
DATA_BLOCK DB3401
TITLE=
VERSION : 0.1

STRUCT
   CM_ID : STRING  [8 ] := '=CSF'; //COMPOSITE MACHINE
   STATION_ID : STRING  [8 ] := '++OP40'; //STATION - TRATTO - ZONE
   ELEMENT_ID : STRING  [8 ] := '+CAB0'; //ELEMENT
   DB_ID : INT := 0 ; //DB SIZE OR TYPE
   PART_STYLE : STRING  [12 ]; //PART STYLE ON LAST STATION
   ACT_CYCLE_TIME : INT ; //ACTUAL CYCLE TIME FOR THIS STYLE
   COUNT_GOOD : INT ; //COUNTER GOOD PIECES
   COUNT_SCRAP : INT ; //COUNTER SCRAP PIECES
   SPARE_00 : ARRAY  [0 .. 15 ] OF //SPARE INTEGER
   INT ;
   SPARE_01 : ARRAY  [0 .. 17 ] OF //SPARE INTEGER
   INT ;
   CODE_EVENT : ARRAY  [0 .. 7 ] OF //CODE EVENT - EXTENDED FAULT CODE DIAGNOSTIC
   INT ;
   EVENT : STRUCT
E0000 : BOOL ; //+CAB0-0ESP10_Q1; 0ESP10_Q1;1
E0001 : BOOL ; //+CAB0-0ESP10_Q2; 0ESP10_Q2;1
E0002 : BOOL ; //+CAB0-0ESP10_0F1; 0ESP10_0F1;1
E0003 : BOOL ; //+CAB0-0ESP10_0F2; 0ESP10_0F2;1
E0004 : BOOL ; //+CAB0-0ESP10_0F3; 0ESP10_0F3;1
E0005 : BOOL ; //+CAB0-0DC43_Q1; 0DC43_Q1;1
E0006 : BOOL ; //+CAB0-0DC43_F1; 0DC43_F1;1
E0007 : BOOL ; //+CAB0-0DC44_UPS; 0DC44_UPS;1
E0008 : BOOL ; //+CAB0-0DC44_0F1; 0DC44_0F1;1
E0009 : BOOL ; //+CAB0-0DP58_A1; 0DP58_A1;1
E0010 : BOOL ; //+CAB0-0EN64_S1F; 0EN64_S1F;1
E0011 : BOOL ; //+CAB0-0FIP65_Q1; 0FIP65_Q1;1
E0012 : BOOL ; //+CAB0-0SPS90_A1; 0SPS90_A1;1
E0013 : BOOL ; //+CAB0-0SPS91_D1; 0SPS91_D1;1
E0014 : BOOL ; //+CAB0-0SPS92_A1; 0SPS92_A1;1
E0015 : BOOL ; //+CAB0-0SPS92_A2; 0SPS92_A2;1
E0016 : BOOL ; //+CAB0-0SPS93_A1; 0SPS93_A1;1
E0017 : BOOL ; //+CAB0-0SPS93_A2; 0SPS93_A2;1
E0018 : BOOL ; //+CAB0-0SPS93_A3; 0SPS93_A3;1
E0019 : BOOL ; //+CAB0-0SPS93_A4; 0SPS93_A4;1
E0020 : BOOL ; //+CAB0-0SPS93_A5; 0SPS93_A5;1
E0021 : BOOL ; //+CAB0-0SPS93_A6; 0SPS93_A6;1
E0022 : BOOL ; //+CAB0-0SPS93_A7; 0SPS93_A7;1
E0023 : BOOL ; //+CAB0-0SPS93_A8; 0SPS93_A8;1
E0024 : BOOL ; //+CAB0-0SPS93_A9; 0SPS93_A9;1
E0025 : BOOL ;
E0026 : BOOL ;
E0027 : BOOL ;
E0028 : BOOL ;
E0029 : BOOL ;
E0030 : BOOL ;
E0031 : BOOL ;
E0032 : BOOL ;
E0033 : BOOL ;
E0034 : BOOL ;
E0035 : BOOL ;
E0036 : BOOL ;
E0037 : BOOL ;
E0038 : BOOL ;
E0039 : BOOL ;
E0040 : BOOL ;
E0041 : BOOL ;
E0042 : BOOL ;
E0043 : BOOL ;
E0044 : BOOL ;
E0045 : BOOL ;
E0046 : BOOL ;
E0047 : BOOL ;
E0048 : BOOL ;
E0049 : BOOL ;
E0050 : BOOL ;
E0051 : BOOL ;
E0052 : BOOL ;
E0053 : BOOL ;
E0054 : BOOL ;
E0055 : BOOL ;
E0056 : BOOL ;
E0057 : BOOL ;
E0058 : BOOL ;
E0059 : BOOL ;
E0060 : BOOL ;
E0061 : BOOL ;
E0062 : BOOL ;
E0063 : BOOL ;
   END_STRUCT;
END_STRUCT;
BEGIN
CM_ID := '=CSF';
STATION_ID := '++OP40';
ELEMENT_ID := '+CAB0';
DB_ID := 0 ;
PART_STYLE := '';
ACT_CYCLE_TIME := 0;
COUNT_GOOD := 0;
COUNT_SCRAP := 0;
SPARE_00[0] := 0;
SPARE_00[1] := 0;
SPARE_00[2] := 0;
SPARE_00[3] := 0;
SPARE_00[4] := 0;
SPARE_00[5] := 0;
SPARE_00[6] := 0;
SPARE_00[7] := 0;
SPARE_00[8] := 0;
SPARE_00[9] := 0;
SPARE_00[10] := 0;
SPARE_00[11] := 0;
SPARE_00[12] := 0;
SPARE_00[13] := 0;
SPARE_00[14] := 0;
SPARE_00[15] := 0;
SPARE_01[0] := 0;
SPARE_01[1] := 0;
SPARE_01[2] := 0;
SPARE_01[3] := 0;
SPARE_01[4] := 0;
SPARE_01[5] := 0;
SPARE_01[6] := 0;
SPARE_01[7] := 0;
SPARE_01[8] := 0;
SPARE_01[9] := 0;
SPARE_01[10] := 0;
SPARE_01[11] := 0;
SPARE_01[12] := 0;
SPARE_01[13] := 0;
SPARE_01[14] := 0;
SPARE_01[15] := 0;
SPARE_01[16] := 0;
SPARE_01[17] := 0;
CODE_EVENT[0] := 0;
CODE_EVENT[1] := 0;
CODE_EVENT[2] := 0;
CODE_EVENT[3] := 0;
CODE_EVENT[4] := 0;
CODE_EVENT[5] := 0;
CODE_EVENT[6] := 0;
CODE_EVENT[7] := 0;
EVENT.E0000 := FALSE;
EVENT.E0001 := FALSE;
EVENT.E0002 := FALSE;
EVENT.E0003 := FALSE;
EVENT.E0004 := FALSE;
EVENT.E0005 := FALSE;
EVENT.E0006 := FALSE;
EVENT.E0007 := FALSE;
EVENT.E0008 := FALSE;
EVENT.E0009 := FALSE;
EVENT.E0010 := FALSE;
EVENT.E0011 := FALSE;
EVENT.E0012 := FALSE;
EVENT.E0013 := FALSE;
EVENT.E0014 := FALSE;
EVENT.E0015 := FALSE;
EVENT.E0016 := FALSE;
EVENT.E0017 := FALSE;
EVENT.E0018 := FALSE;
EVENT.E0019 := FALSE;
EVENT.E0020 := FALSE;
EVENT.E0021 := FALSE;
EVENT.E0022 := FALSE;
EVENT.E0023 := FALSE;
EVENT.E0024 := FALSE;
EVENT.E0025 := FALSE;
EVENT.E0026 := FALSE;
EVENT.E0027 := FALSE;
EVENT.E0028 := FALSE;
EVENT.E0029 := FALSE;
EVENT.E0030 := FALSE;
EVENT.E0031 := FALSE;
EVENT.E0032 := FALSE;
EVENT.E0033 := FALSE;
EVENT.E0034 := FALSE;
EVENT.E0035 := FALSE;
EVENT.E0036 := FALSE;
EVENT.E0037 := FALSE;
EVENT.E0038 := FALSE;
EVENT.E0039 := FALSE;
EVENT.E0040 := FALSE;
EVENT.E0041 := FALSE;
EVENT.E0042 := FALSE;
EVENT.E0043 := FALSE;
EVENT.E0044 := FALSE;
EVENT.E0045 := FALSE;
EVENT.E0046 := FALSE;
EVENT.E0047 := FALSE;
EVENT.E0048 := FALSE;
EVENT.E0049 := FALSE;
EVENT.E0050 := FALSE;
EVENT.E0051 := FALSE;
EVENT.E0052 := FALSE;
EVENT.E0053 := FALSE;
EVENT.E0054 := FALSE;
EVENT.E0055 := FALSE;
EVENT.E0056 := FALSE;
EVENT.E0057 := FALSE;
EVENT.E0058 := FALSE;
EVENT.E0059 := FALSE;
EVENT.E0060 := FALSE;
EVENT.E0061 := FALSE;
EVENT.E0062 := FALSE;
EVENT.E0063 := FALSE;
END_DATA_BLOCK
